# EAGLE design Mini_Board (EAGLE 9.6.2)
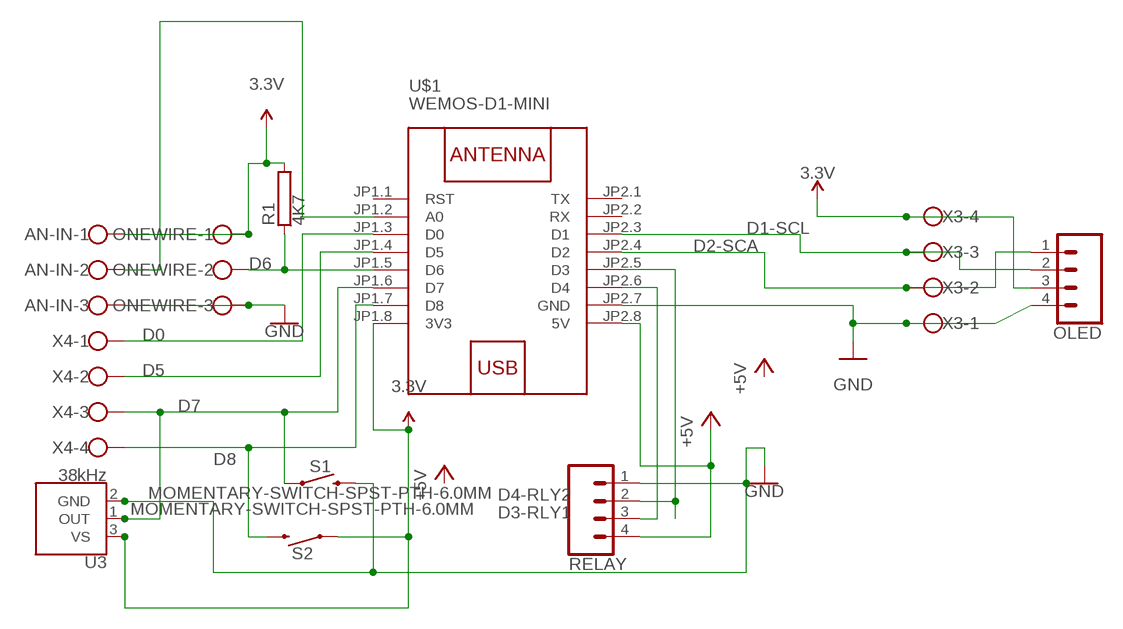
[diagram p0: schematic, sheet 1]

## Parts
AN-IN  W237-103  [W237-103]
OLED  CONN_04PTH  [1X04]
ONEWIRE  W237-103  [W237-103]
R1  4K7  RRS1/4  [RS1/4]
RELAY  CONN_04PTH  [1X04]
S1  MOMENTARY-SWITCH-SPST-PTH-6.0MM  [TACTILE_SWITCH_PTH_6.0MM]
S2  MOMENTARY-SWITCH-SPST-PTH-6.0MM  [TACTILE_SWITCH_PTH_6.0MM]
U3  38kHz  TSOP38238  [TSOP382]
U$1  WEMOS-D1-MINI  [WEMOS-D1-MINI]
X3  W237-4  [W237-4]
X4  W237-4  [W237-4]

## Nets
3.3V: AN-IN.1 OLED.3 ONEWIRE.1 R1.2 S2.1 U3.3(VS) U$1.JP1.8(3V3) X3.4
+5V: RELAY.4 U$1.JP2.8(5V)
D0: U$1.JP1.3(D0) X4.1
D1-SCL: OLED.2 U$1.JP2.3(D1) X3.3
D2-SCA: OLED.1 U$1.JP2.4(D2) X3.2
D3-RLY1: RELAY.2 U$1.JP2.5(D3)
D4-RLY2: RELAY.3 U$1.JP2.6(D4)
D5: U$1.JP1.4(D5) X4.2
D6: ONEWIRE.2 R1.1 U$1.JP1.5(D6)
D7: S1.1 U3.1(OUT) U$1.JP1.6(D7) X4.3
D8: S2.3 U$1.JP1.7(D8) X4.4
GND: AN-IN.3 OLED.4 ONEWIRE.3 RELAY.1 S1.3 U3.2(GND) U$1.JP2.7(GND) X3.1
N$7: AN-IN.2 U$1.JP1.2(A0)
Unconnected: U$1.JP1.1(RST) U$1.JP2.1(TX) U$1.JP2.2(RX)

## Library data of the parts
AN-IN ONEWIRE = con-wago-500:W237-103: WAGO SCREW CLAMP; MPN: 237-103; OC_FARNELL: unknown; OC_NEWARK: 18M7116
OLED RELAY = SparkFun-Connectors:CONN_04: Multi connection point. Often used as Generic Header-pin footprint for 0.1 inch spaced/style header connections On any of the 0.1 inch spaced packages, you can populate with these: Break Away Headers - Straight (PRT-00116) Break Away Male Headers - Right Angle (PRT-00553) Female Headers (PRT-00115)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; PROD_ID: CONN-09696
R1 = resistor-power:R: Power Resitor; MF: OHMITE; MPN: RRS1K0; OC_FARNELL: unknown; OC_NEWARK: 01F7661
S1 S2 = SparkFun-Switches:MOMENTARY-SWITCH-SPST: Momentary Switch (Pushbutton) - SPST; PROD_ID: SWCH-08441; SF_SKU: COM-00097
U3 = SparkFun-Sensors:TSOP382: Vishay Semiconductor TSOP32838 - 38kHz IR Receiver These products are miniaturized IR receiver modules for infrared remote control systems. A PIN diode and a preamplifier are assembled on a leadframe, the epoxy package contains an IR filter. The demodulated output signal can be directly connected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; PROD_ID: SEN-10266
U$1 = diy-modules:WEMOS-D1-MINI: WEMOS D1 mini: Mini Wi-Fi Board based on ESP-8266 device More details can be found here: https://www.wemos.cc/product/d1-mini.html Click here to find device on ebay.com
X3 X4 = con-wago-500:W237-4: WAGO SCREW CLAMP; OC_FARNELL: unknown; OC_NEWARK: unknown

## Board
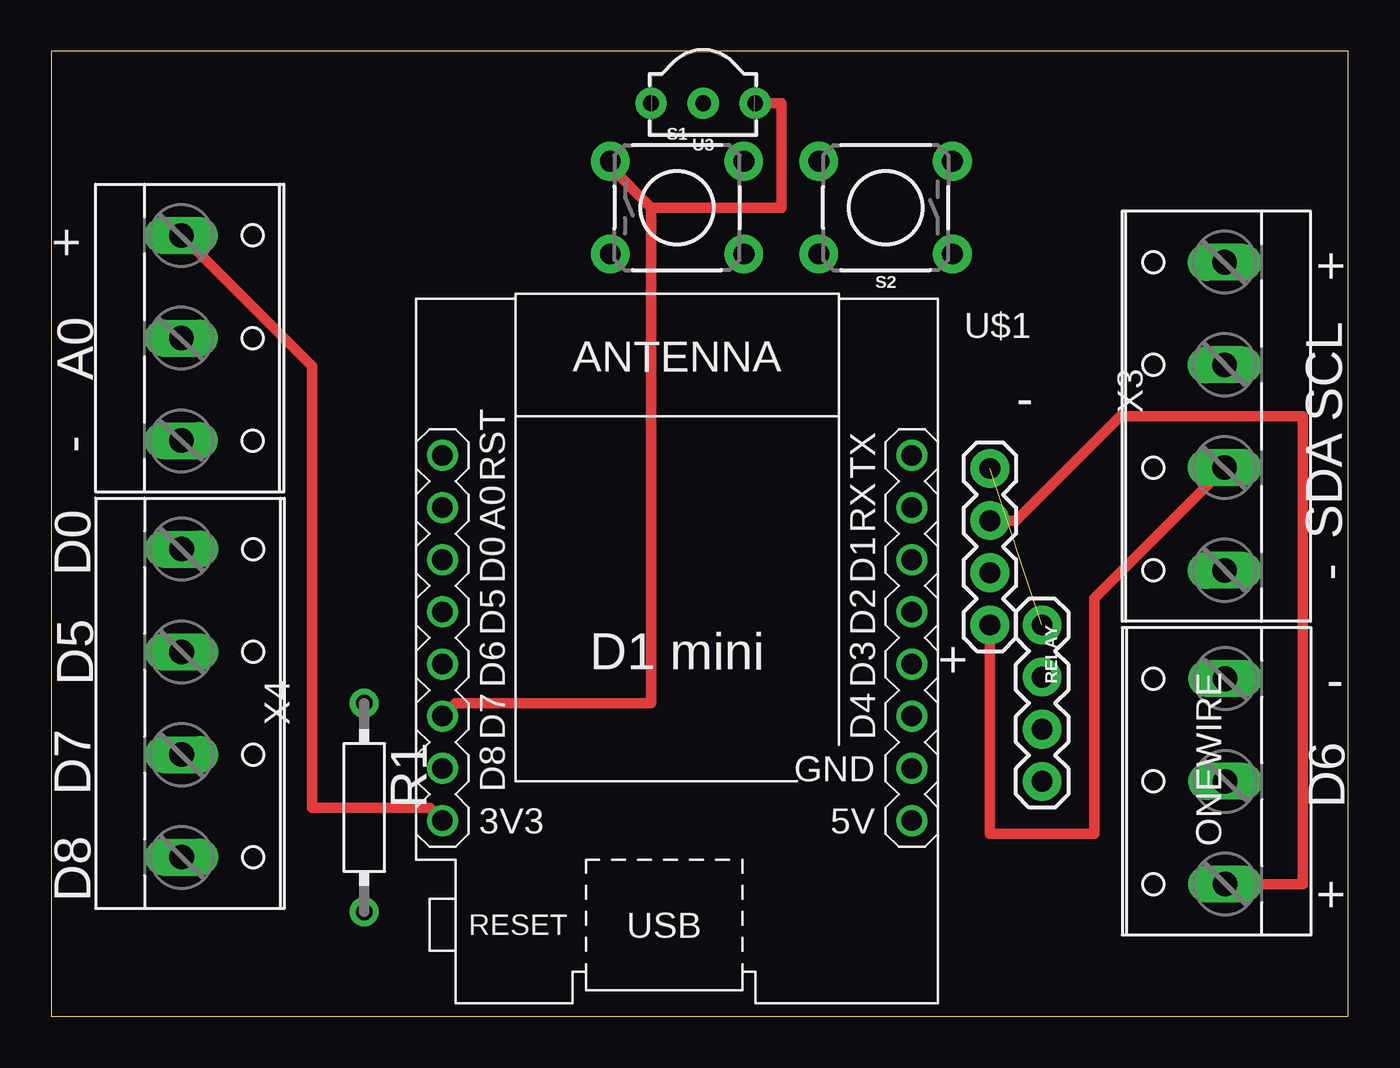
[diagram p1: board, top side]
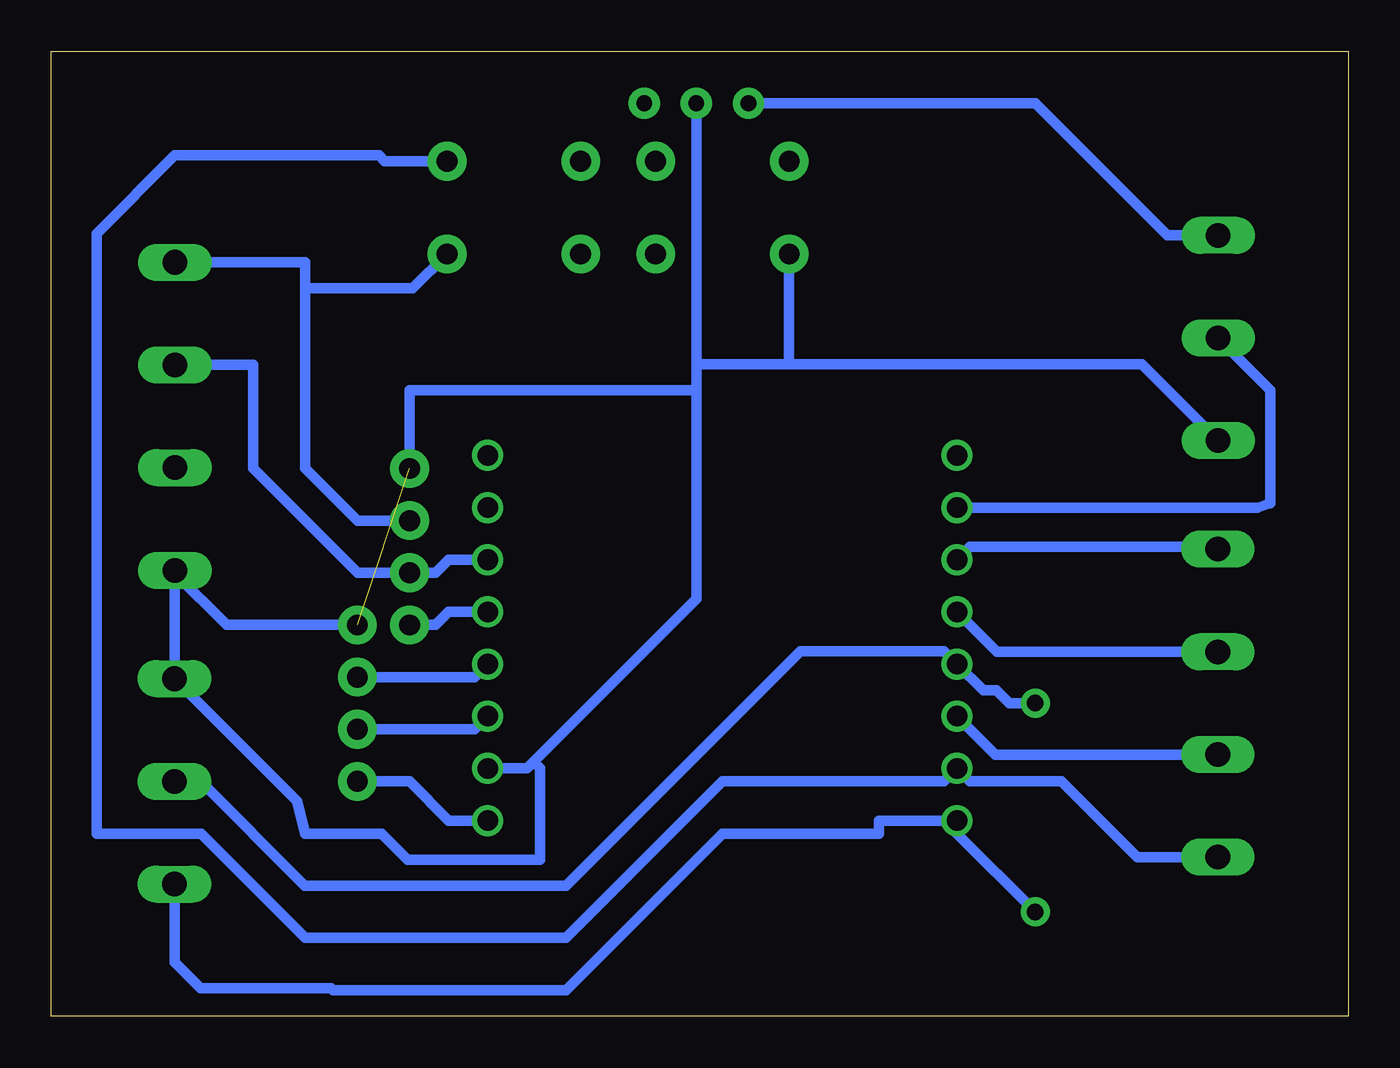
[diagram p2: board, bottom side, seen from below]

Size 63.17 x 46.98 mm. Coordinates in mm from the lower left corner, seen from the top.
Outline: 0,0 63.17,0 63.17,46.98 0,46.98 0,0
Copper layers (1*16): Top 0.035mm / dielectric 1.5mm / Bottom 0.035mm
Design rules "default": minimum track width 6mil, minimum drill 0.35mm, track to track 6mil, track to pad 6mil, pad to pad 6mil, via to via 6mil, smd to smd 6mil, copper to edge 40mil, drill to drill 6mil, minimum pad ring 10mil, minimum via ring 8mil, stop-mask expansion 4mil, vias tented up to drill 0mil, thermal gap 10mil

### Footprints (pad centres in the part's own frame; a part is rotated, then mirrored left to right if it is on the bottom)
W237-103 = drill 1.194 long: 1 -5,-1.29; 2 0,-1.29; 3 5,-1.29
1X04 = drill 1.016 pad 1.88: 1 0,0; 2 2.54,0; 3 5.08,0; 4 7.62,0
RS1/4 = drill 0.8 pad 1.4: 1 -5.08,0; 2 5.08,0
TACTILE_SWITCH_PTH_6.0MM = drill 1.016 pad 1.88: 1 -3.251,2.261; 2 3.251,2.261; 3 -3.251,-2.261; 4 3.251,-2.261
TSOP382 = drill 0.762 pad 1.524: 1 -2.54,0; 2 0,0; 3 2.54,0
WEMOS-D1-MINI = drill 1: JP1.1 -11.43,9.525; JP1.2 -11.43,6.985; JP1.3 -11.43,4.445; JP1.4 -11.43,1.905; JP1.5 -11.43,-0.635; JP1.6 -11.43,-3.175; JP1.7 -11.43,-5.715; JP1.8 -11.43,-8.255; JP2.1 11.43,9.525; JP2.2 11.43,6.985; JP2.3 11.43,4.445; JP2.4 11.43,1.905; JP2.5 11.43,-0.635; JP2.6 11.43,-3.175; JP2.7 11.43,-5.715; JP2.8 11.43,-8.255
W237-4 = drill 1.194 long: 1 -7.5,-1.27; 2 -2.5,-1.27; 3 2.5,-1.27; 4 7.5,-1.27

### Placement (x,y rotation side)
AN-IN  7.62,33.02 270 top
OLED  45.72,19.05 90 top
ONEWIRE  55.88,11.43 90 top
R1  15.24,10.16 270 top
RELAY  48.26,19.05 270 top
S1  30.48,39.37 0 top
S2  40.64,39.37 180 top
U3  31.75,44.45 180 top
U$1  30.48,17.78 0 top
X3  55.88,29.21 90 top
X4  7.62,15.24 270 top

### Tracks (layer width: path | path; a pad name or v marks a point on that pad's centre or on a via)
3.3V
  Top 0.508: OLED.3 46.99,24.13 52.07,29.21 60.96,29.21 60.96,6.43 ONEWIRE.1 | AN-IN.1 12.7,31.65 12.7,10.16 18.41,10.16 U$1.JP1.8
  Bottom 0.508: OLED.3 48.26,24.13 50.8,26.67 50.8,35.44 | 50.8,35.44 50.8,36.71 X3.4 | ONEWIRE.1 57.17,2.62 55.9,1.35 49.53,1.35 49.45,1.27 38.1,1.27 30.48,8.89 22.86,8.89 22.86,9.53 U$1.JP1.8 19.05,8.89 R1.2 | U3.3 15.24,44.45 8.81,38.02 AN-IN.1 | 50.8,35.44 45.56,35.44 S2.1
+5V
  Bottom 0.508: U$1.JP2.8 43.81,9.53 45.72,11.43 RELAY.4
D0
  Bottom 0.508: U$1.JP1.3 18.41,22.86 6.47,22.86 X4.1
D1-SCL
  Bottom 0.508: X3.3 53.34,31.71 53.34,26.67 48.26,21.59 OLED.2 44.45,21.59 43.81,22.23 U$1.JP2.3
D2-SCA
  Top 0.508: X3.2 50.8,20.36 50.8,8.89 45.72,8.89 OLED.1
  Bottom 0.508: OLED.1 44.45,19.05 43.81,19.68 U$1.JP2.4
D3-RLY1
  Bottom 0.508: U$1.JP2.5 42.55,16.51 RELAY.2
D4-RLY2
  Bottom 0.508: U$1.JP2.6 42.55,13.97 RELAY.3
D5
  Bottom 0.508: U$1.JP1.4 17.11,17.74 X4.2
D6
  Bottom 0.508: ONEWIRE.2 55.9,11.43 50.82,6.35 38.1,6.35 26.67,17.78 19.68,17.78 U$1.JP1.5 17.78,15.88 17.14,15.88 16.51,15.24 R1.1
D7
  Top 0.508: U$1.JP1.6 19.68,15.24 29.21,15.24 29.22,39.37 | 29.22,39.37 35.55,39.36 35.56,39.37 35.56,44.45 U3.1 | 29.22,39.37 27.23,41.36 S1.1
  Bottom 0.508: U$1.JP1.6 17.18,12.74 X4.3
D8
  Bottom 0.508: X4.4 10.28,7.74 13.97,11.43 18.41,11.43 U$1.JP1.7 19.68,11.43 30.48,11.43 38.1,3.81 50.8,3.81 55.88,8.89 60.96,8.89 60.96,38.1 57.15,41.91 47.21,41.91 46.93,41.63 S2.3
GND  (1 unrouted)
  Top 0.508: AN-IN.3 6.41,27.94
  Bottom 0.508: U$1.JP2.7 40.01,12.06 39.69,12.38 | 39.69,12.38 39.37,12.06 39.37,7.62 45.82,7.62 47.09,8.89 50.8,8.89 51.21,10.47 ONEWIRE.3 57.17,21.59 57.15,21.61 X3.1 57.15,21.57 54.63,19.05 RELAY.1 | OLED.4 45.72,30.48 31.75,30.48 U3.2 | AN-IN.3 10.06,31.75 27.23,31.75 S1.3 | 26.67,31.75 31.75,31.75 31.75,20.32 39.69,12.38
N$7
  Bottom 0.508: U$1.JP1.2 4.42,24.77 3.79,24.97 3.79,30.48 AN-IN.2

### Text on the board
tNames: + | + | A0 | - | SCL | - | SDA | D0 | - | + | D5 | - | D7 | D6 | D8 | +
